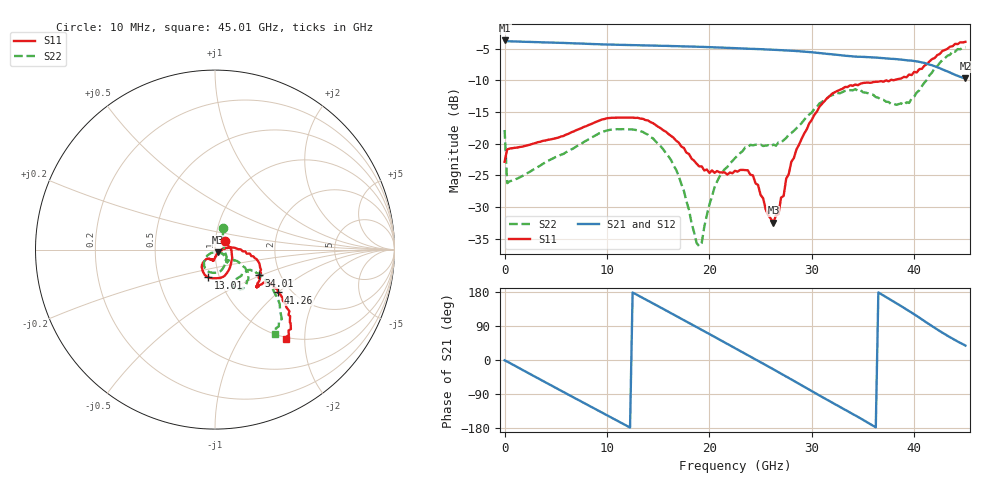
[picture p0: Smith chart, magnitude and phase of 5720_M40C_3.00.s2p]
! Device:  ADRF5720
! Description: 0.5dB LSB GaAs MMIC 6-bit Digital Attenuator
! Frequency:  0.000009 -  40 GHz
! Ports:
!	RF1	= Port 1
!	RF2	= Port 2
! Vdd:  3.3 Volt
! Vss:  -3.3 Volt
! Control:  0/3.3 Volt
! State:  3.00 dB attenuation
! Data:  The device was measured using G-S-G Probes on a matrix board.
!  Data was collected using an calibrated 4 port network analyzer.
!  The reference plane for this measurement is at the launchers.
! Note:  Analog Devices supplies this data as a sample of measured data
!  for this product.  Your particular data for this product may vary.
!  Data was taken at -40 degrees C.
!  Analog Devices reserves the right to change this data at anytime.
# GHZ S DB R 45.0
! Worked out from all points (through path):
!   181 points, 10 MHz to 45.01 GHz, reference 45 ohm
!   highest |S21| = -3.73 dB at 10 MHz (marker M1); lowest = -9.7 dB at 45.01 GHz (marker M2)
!   group delay of S21, straight-line fit = 41.8 ps
!   lowest |S11| = -32.5 dB at 26.26 GHz (marker M3), VSWR 1.05, Z = 46.7 - j1.38 ohm
!   |S11| at or under -10 dB: start of sweep to 37.69 GHz; 37.97875 GHz to 38.02923 GHz (50.48 MHz wide, 0.133 % of centre)
!   |S22| runs from -36.2 to -4.8 dB; largest |S21 - S12| = 0.0024
!   S11 on the Smith chart (normalised r, x): 10 MHz: 1.11, +0.10; 13.01 GHz: 0.88, -0.28; 34.01 GHz: 1.56, -0.49; 41.26 GHz: 1.71, -1.00; 45.01 GHz: 0.97, -1.62
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0.01  -22.88 40.8  -3.73 -0.9  -3.75 -0.9  -17.86 70.6
0.26  -20.92 1.0  -3.85 -4.0  -3.87 -4.1  -26.25 3.2
2.01  -20.38 -13.6  -3.94 -29.9  -3.96 -29.9  -24.87 -15.5
4.26  -19.40 -26.3  -4.05 -62.7  -4.07 -62.7  -22.72 -29.5
7.76  -17.37 -54.3  -4.24 -113.5  -4.25 -113.5  -19.74 -59.0
10.51  -15.93 -77.9  -4.40 -153.1  -4.42 -153.1  -17.79 -84.2
13.01  -15.94 -103.8  -4.50 171.0  -4.52 170.9  -17.93 -109.4
15.26  -17.59 -122.5  -4.57 138.3  -4.58 138.2  -20.46 -130.4
17.01  -19.84 -132.4  -4.64 112.7  -4.65 112.6  -25.11 -142.2
19.01  -23.60 -129.9  -4.73 83.2  -4.75 83.2  -36.20 -79.6
20.51  -24.62 -114.0  -4.82 61.1  -4.84 61.0  -26.91 -26.8
22.76  -24.44 -103.9  -4.96 27.8  -4.98 27.7  -21.90 -41.0
24.26  -25.03 -95.6  -5.06 5.5  -5.08 5.4  -20.28 -47.1
26.26  -32.49 -38.4  -5.20 -24.7  -5.21 -24.8  -20.16 -38.1
26.76  -31.14 -9.9  -5.25 -32.2  -5.26 -32.4  -19.82 -35.4
28.01  -22.88 7.0  -5.35 -51.2  -5.37 -51.4  -18.35 -30.0
30.26  -15.47 -3.5  -5.63 -86.0  -5.65 -86.1  -14.52 -31.0
34.01  -10.88 -30.3  -6.24 -142.8  -6.27 -142.9  -11.61 -52.2
37.76  -9.93 -40.5  -6.63 158.2  -6.65 158.1  -13.78 -60.1
39.51  -9.11 -32.1  -6.89 129.4  -6.91 129.2  -13.59 -33.6
41.26  -7.45 -34.2  -7.41 98.2  -7.43 98.0  -9.93 -30.3
45.01  -3.95 -51.5  -9.71 38.1  -9.74 38.0  -4.80 -54.7
